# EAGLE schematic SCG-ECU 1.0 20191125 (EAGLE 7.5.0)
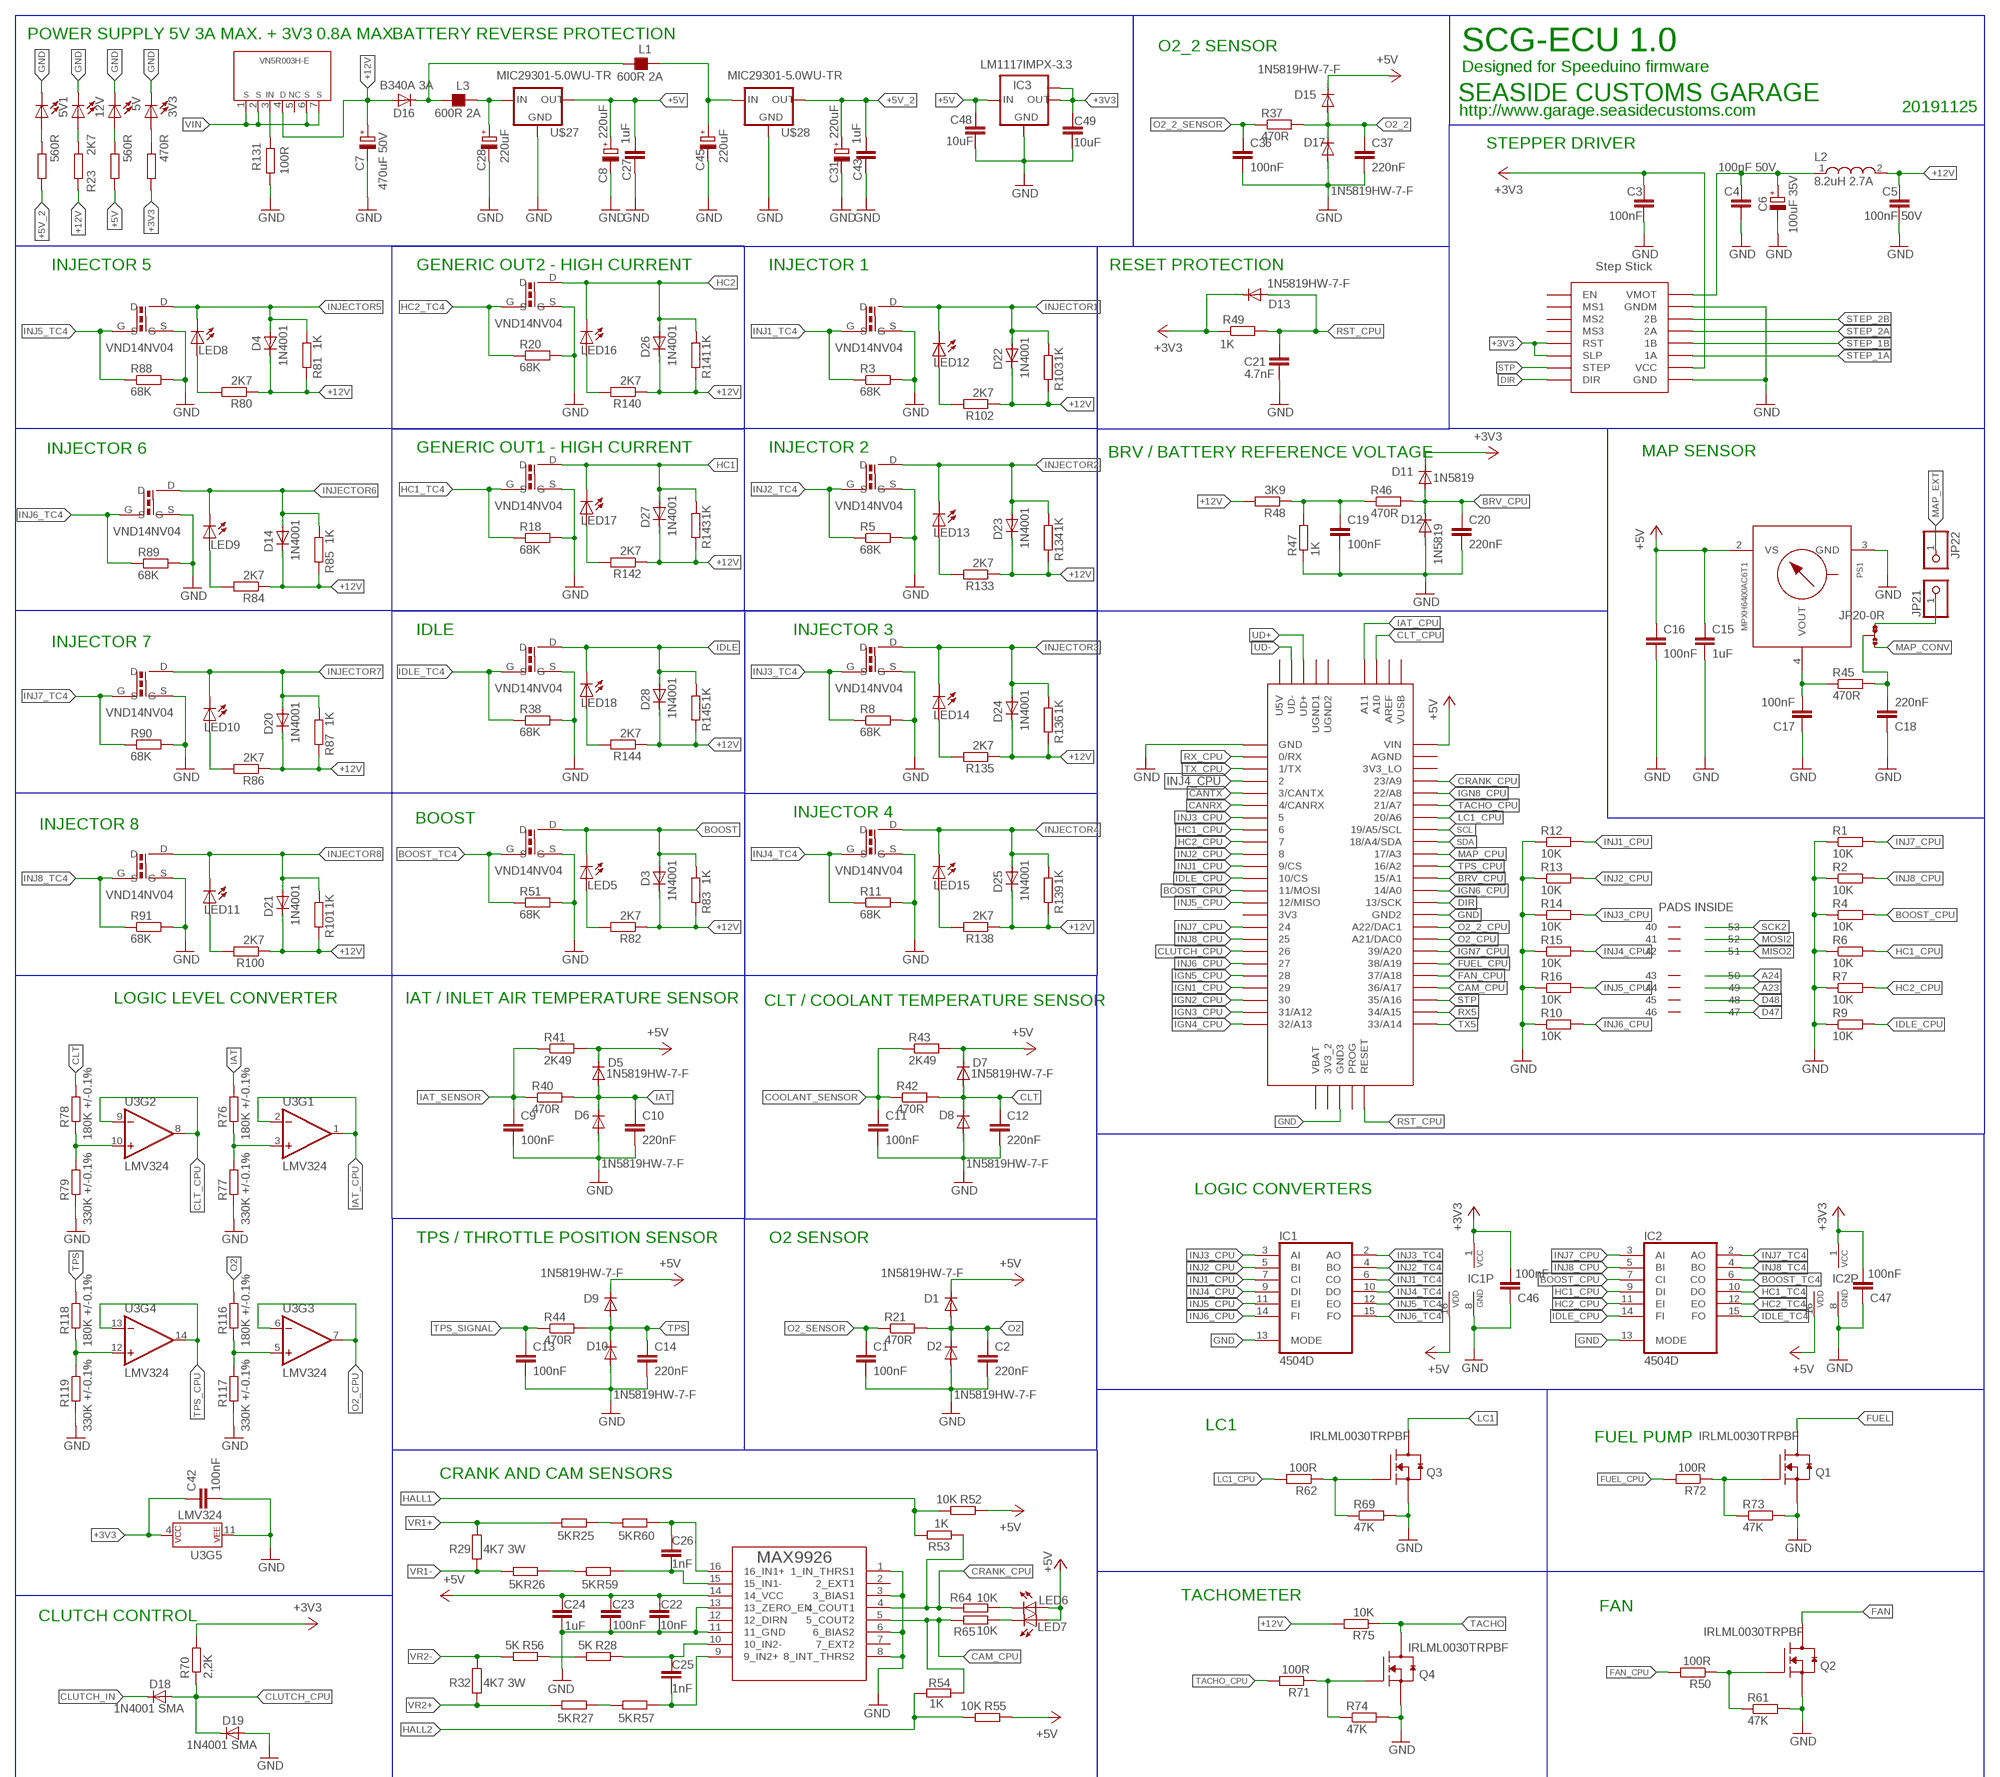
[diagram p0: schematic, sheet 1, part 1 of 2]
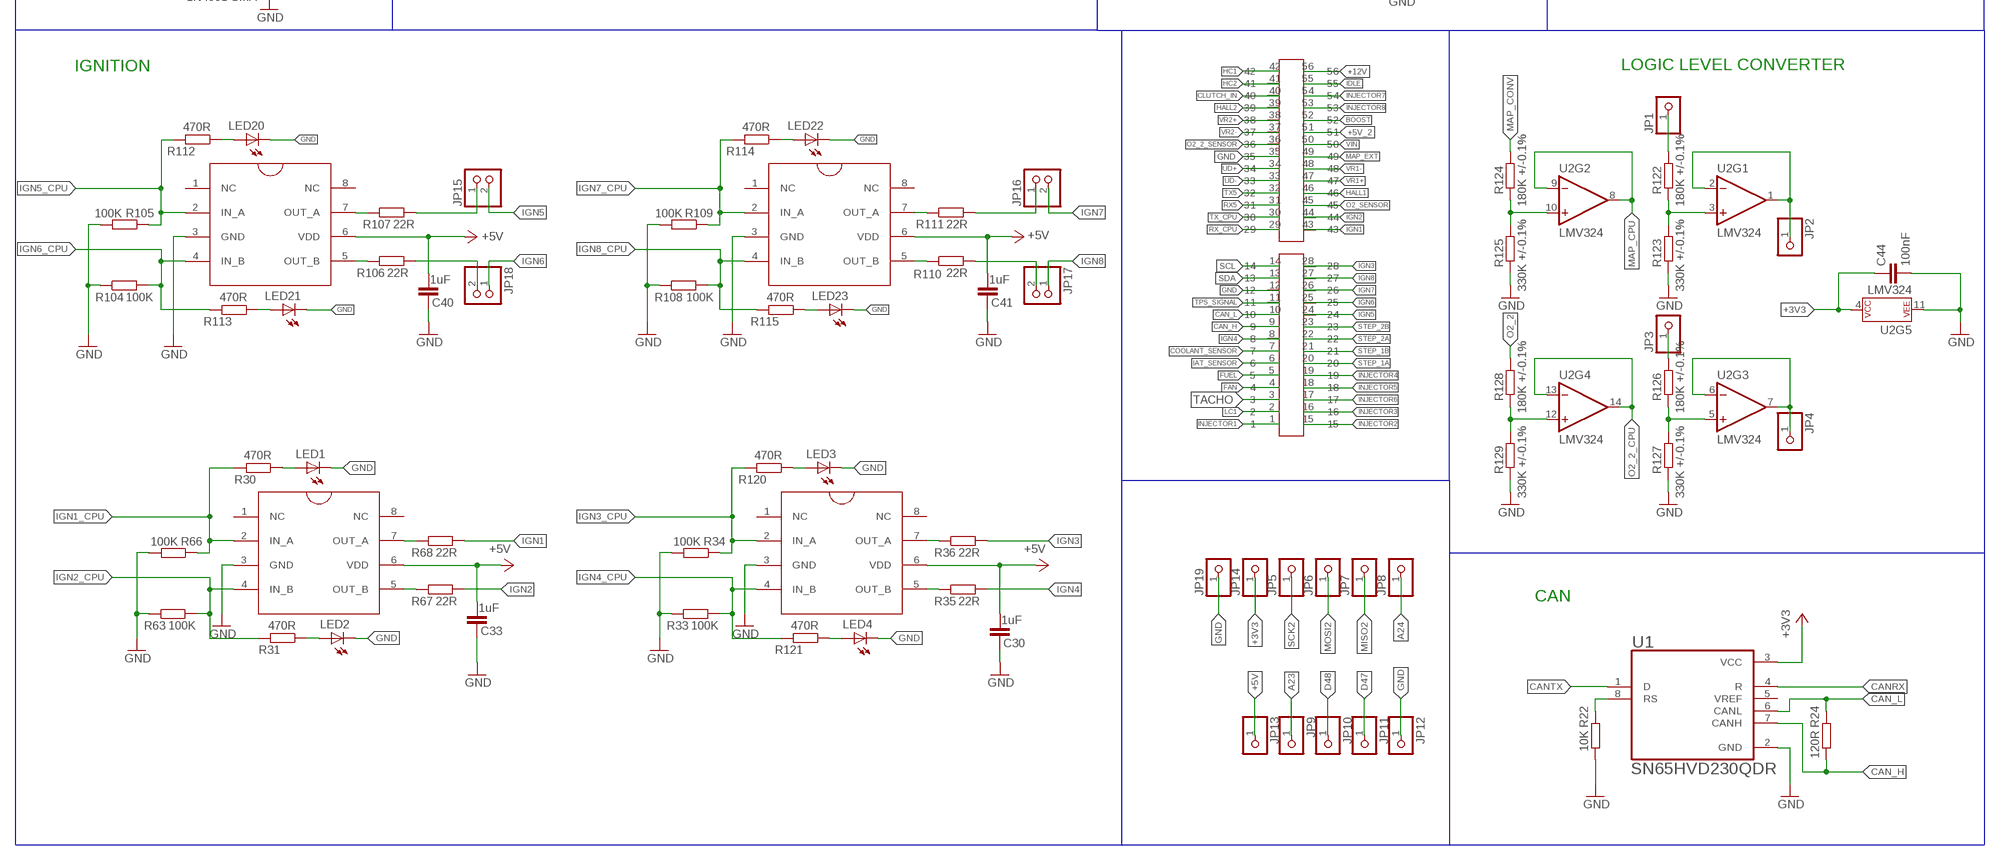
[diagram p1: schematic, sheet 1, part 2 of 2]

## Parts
3V3  LEDCHIP-LED0805  [CHIP-LED0805]
5V  LEDCHIP-LED0805  [CHIP-LED0805]
5V1  LEDCHIP-LED0805  [CHIP-LED0805]
12V  LEDCHIP-LED0805  [CHIP-LED0805]
C1  100nF  C-EUC0805  [C0805]
C2  220nF  C-EUC0805  [C0805]
C3  100nF  C-EUC0805  [C0805]
C4  100nF 50V  C-EUC0805  [C0805]
C5  100nF 50V  C-EUC0805  [C0805]
C6  100uF 35V  CPOL-EUD  [PANASONIC_D]
C7  470uF 50V  CPOL-EUG  [PANASONIC_G]
C8  220uF  CPOL-EUD  [PANASONIC_D]
C9  100nF  C-EUC0805  [C0805]
C10  220nF  C-EUC0805  [C0805]
C11  100nF  C-EUC0805  [C0805]
C12  220nF  C-EUC0805  [C0805]
C13  100nF  C-EUC0805  [C0805]
C14  220nF  C-EUC0805  [C0805]
C15  1uF  C-EUC0805  [C0805]
C16  100nF  C-EUC0805  [C0805]
C17  100nF  C-EUC0805  [C0805]
C18  220nF  C-EUC0805  [C0805]
C19  100nF  C-EUC0805  [C0805]
C20  220nF  C-EUC0805  [C0805]
C21  4.7nF  C-EUC0805  [C0805]
C22  10nF  C-EUC0805  [C0805]
C23  100nF  C-EUC0805  [C0805]
C24  1uF  C-EUC0805  [C0805]
C25  1nF  C-EUC0805  [C0805]
C26  1nF  C-EUC0805  [C0805]
C27  1uF  C-EUC0805  [C0805]
C28  220uF  CPOL-EUD  [PANASONIC_D]
C30  1uF  C-EUC0805  [C0805]
C31  220uF  CPOL-EUD  [PANASONIC_D]
C33  1uF  C-EUC0805  [C0805]
C36  100nF  C-EUC0805  [C0805]
C37  220nF  C-EUC0805  [C0805]
C40  1uF  C-EUC0805  [C0805]
C41  1uF  C-EUC0805  [C0805]
C42  100nF  C-EUC0805  [C0805]
C43  1uF  C-EUC0805  [C0805]
C44  100nF  C-EUC0805  [C0805]
C45  220uF  CPOL-EUD  [PANASONIC_D]
C46  100nF  C-EUC0805  [C0805]
C47  100nF  C-EUC0805  [C0805]
C48  10uF  C-EUC0805  [C0805]
C49  10uF  C-EUC0805  [C0805]
D1  1N5819HW-7-F  DIODE-SOD123  [SOD123]
D2  1N5819HW-7-F  DIODE-SOD123  [SOD123]
D3  1N4001  DIODE-D-2.5  [D-2.5]
D4  1N4001  DIODE-D-2.5  [D-2.5]
D5  1N5819HW-7-F  DIODE-SOD123  [SOD123]
D6  1N5819HW-7-F  DIODE-SOD123  [SOD123]
D7  1N5819HW-7-F  DIODE-SOD123  [SOD123]
D8  1N5819HW-7-F  DIODE-SOD123  [SOD123]
D9  1N5819HW-7-F  DIODE-SOD123  [SOD123]
D10  1N5819HW-7-F  DIODE-SOD123  [SOD123]
D11  1N5819  DIODE-SOD123  [SOD123]
D12  1N5819  DIODE-SOD123  [SOD123]
D13  1N5819HW-7-F  DIODE-SOD123  [SOD123]
D14  1N4001  DIODE-D-2.5  [D-2.5]
D15  1N5819HW-7-F  DIODE-SOD123  [SOD123]
D16  B340A 3A  S1A  [DO214AC]
D17  1N5819HW-7-F  DIODE-SOD123  [SOD123]
D18  1N4001 SMA  S1A  [DO214AC]
D19  1N4001 SMA  S1A  [DO214AC]
D20  1N4001  DIODE-D-2.5  [D-2.5]
D21  1N4001  DIODE-D-2.5  [D-2.5]
D22  1N4001  DIODE-D-2.5  [D-2.5]
D23  1N4001  DIODE-D-2.5  [D-2.5]
D24  1N4001  DIODE-D-2.5  [D-2.5]
D25  1N4001  DIODE-D-2.5  [D-2.5]
D26  1N4001  DIODE-D-2.5  [D-2.5]
D27  1N4001  DIODE-D-2.5  [D-2.5]
D28  1N4001  DIODE-D-2.5  [D-2.5]
IC1  4504D  [SO16]
IC2  4504D  [SO16]
IC3  LM1117IMPX-3.3  [SOT223]
JP1  PINHD-1X1  [1X01]
JP2  PINHD-1X1  [1X01]
JP3  PINHD-1X1  [1X01]
JP4  PINHD-1X1  [1X01]
JP5  PINHD-1X1  [1X01]
JP6  PINHD-1X1  [1X01]
JP7  PINHD-1X1  [1X01]
JP8  PINHD-1X1  [1X01]
JP9  PINHD-1X1  [1X01]
JP10  PINHD-1X1  [1X01]
JP11  PINHD-1X1  [1X01]
JP12  PINHD-1X1  [1X01]
JP13  PINHD-1X1  [1X01]
JP14  PINHD-1X1  [1X01]
JP15  PINHD-1X2  [1X02]
JP16  PINHD-1X2  [1X02]
JP17  PINHD-1X2  [1X02]
JP18  PINHD-1X2  [1X02]
JP19  PINHD-1X1  [1X01]
JP20  0R-JUMPA  [A0R-JMP]
JP21  PINHD-1X1  [1X01]
JP22  PINHD-1X1  [1X01]
L1  600R 2A  FB_1206  [L1206]
L2  8.2uH 2.7A  WE-PD_7332/7345_PLASTIC_BASE  [WE-PD_7332/7345_PLASTIC_BASE]
L3  600R 2A  FB_1206  [L1206]
LED1  LEDCHIP-LED0805  [CHIP-LED0805]
LED2  LEDCHIP-LED0805  [CHIP-LED0805]
LED3  LEDCHIP-LED0805  [CHIP-LED0805]
LED4  LEDCHIP-LED0805  [CHIP-LED0805]
LED5  LEDCHIPLED_0805  [CHIPLED_0805]
LED6  LEDCHIP-LED0805  [CHIP-LED0805]
LED7  LEDCHIP-LED0805  [CHIP-LED0805]
LED8  LEDCHIPLED_0805  [CHIPLED_0805]
LED9  LEDCHIPLED_0805  [CHIPLED_0805]
LED10  LEDCHIPLED_0805  [CHIPLED_0805]
LED11  LEDCHIPLED_0805  [CHIPLED_0805]
LED12  LEDCHIPLED_0805  [CHIPLED_0805]
LED13  LEDCHIPLED_0805  [CHIPLED_0805]
LED14  LEDCHIPLED_0805  [CHIPLED_0805]
LED15  LEDCHIPLED_0805  [CHIPLED_0805]
LED16  LEDCHIPLED_0805  [CHIPLED_0805]
LED17  LEDCHIPLED_0805  [CHIPLED_0805]
LED18  LEDCHIPLED_0805  [CHIPLED_0805]
LED20  LEDCHIP-LED0805  [CHIP-LED0805]
LED21  LEDCHIP-LED0805  [CHIP-LED0805]
LED22  LEDCHIP-LED0805  [CHIP-LED0805]
LED23  LEDCHIP-LED0805  [CHIP-LED0805]
PS1  MPXH6400AC6T1  [1317A]
Q1  IRLML0030TRPBF  MOSFET-NCH_SOT-23  [SOT95P280X135-3N]
Q2  IRLML0030TRPBF  MOSFET-NCH_SOT-23  [SOT95P280X135-3N]
Q3  IRLML0030TRPBF  MOSFET-NCH_SOT-23  [SOT95P280X135-3N]
Q4  IRLML0030TRPBF  MOSFET-NCH_SOT-23  [SOT95P280X135-3N]
R1  10K  R-EU_R0805  [R0805]
R2  10K  R-EU_R0805  [R0805]
R3  68K  R-EU_R0805  [R0805]
R4  10K  R-EU_R0805  [R0805]
R5  68K  R-EU_R0805  [R0805]
R6  10K  R-EU_R0805  [R0805]
R7  10K  R-EU_R0805  [R0805]
R8  68K  R-EU_R0805  [R0805]
R9  10K  R-EU_R0805  [R0805]
R10  10K  R-EU_R0805  [R0805]
R11  68K  R-EU_R0805  [R0805]
R12  10K  R-EU_R0805  [R0805]
R13  10K  R-EU_R0805  [R0805]
R14  10K  R-EU_R0805  [R0805]
R15  10K  R-EU_R0805  [R0805]
R16  10K  R-EU_R0805  [R0805]
R18  68K  R-EU_R0805  [R0805]
R20  68K  R-EU_R0805  [R0805]
R21  470R  R-EU_R0805  [R0805]
R22  10K  R-EU_R0805  [R0805]
R23  2K7  R-EU_R0805  [R0805]
R24  120R  R-EU_R0805  [R0805]
R25  5K  R-EU_R0805  [R0805]
R26  5K  R-EU_R0805  [R0805]
R27  5K  R-EU_R0805  [R0805]
R28  5K  R-EU_R0805  [R0805]
R29  4K7 3W  R-EU_R2512  [R2512]
R30  470R  R-EU_R0805  [R0805]
R31  470R  R-EU_R0805  [R0805]
R32  4K7 3W  R-EU_R2512  [R2512]
R33  100K  R-EU_R0805  [R0805]
R34  100K  R-EU_R0805  [R0805]
R35  22R  R-EU_M1206  [M1206]
R36  22R  R-EU_M1206  [M1206]
R37  470R  R-EU_R0805  [R0805]
R38  68K  R-EU_R0805  [R0805]
R40  470R  R-EU_R0805  [R0805]
R41  2K49  R-EU_R0805  [R0805]
R42  470R  R-EU_R0805  [R0805]
R43  2K49  R-EU_R0805  [R0805]
R44  470R  R-EU_R0805  [R0805]
R45  470R  R-EU_R0805  [R0805]
R46  470R  R-EU_R0805  [R0805]
R47  1K  R-EU_R0805  [R0805]
R48  3K9  R-EU_R0805  [R0805]
R49  1K  R-EU_R0805  [R0805]
R50  100R  R-EU_R0805  [R0805]
R51  68K  R-EU_R0805  [R0805]
R52  10K  R-EU_R0805  [R0805]
R53  1K  R-EU_R0805  [R0805]
R54  1K  R-EU_R0805  [R0805]
R55  10K  R-EU_R0805  [R0805]
R56  5K  R-EU_R0805  [R0805]
R57  5K  R-EU_R0805  [R0805]
R59  5K  R-EU_R0805  [R0805]
R60  5K  R-EU_R0805  [R0805]
R61  47K  R-EU_R0805  [R0805]
R62  100R  R-EU_R0805  [R0805]
R63  100K  R-EU_R0805  [R0805]
R64  10K  R-EU_R0805  [R0805]
R65  10K  R-EU_R0805  [R0805]
R66  100K  R-EU_R0805  [R0805]
R67  22R  R-EU_M1206  [M1206]
R68  22R  R-EU_M1206  [M1206]
R69  47K  R-EU_R0805  [R0805]
R70  2,2K  R-EU_R0805  [R0805]
R71  100R  R-EU_R0805  [R0805]
R72  100R  R-EU_R0805  [R0805]
R73  47K  R-EU_R0805  [R0805]
R74  47K  R-EU_R0805  [R0805]
R75  10K  R-EU_R0805  [R0805]
R76  180K +/-0.1%  R-EU_R0805  [R0805]
R77  330K +/-0.1%  R-EU_R0805  [R0805]
R78  180K +/-0.1%  R-EU_R0805  [R0805]
R79  330K +/-0.1%  R-EU_R0805  [R0805]
R80  2K7  R-EU_R0805  [R0805]
R81  1K  R-EU_R0805  [R0805]
R82  2K7  R-EU_R0805  [R0805]
R83  1K  R-EU_R0805  [R0805]
R84  2K7  R-EU_R0805  [R0805]
R85  1K  R-EU_R0805  [R0805]
R86  2K7  R-EU_R0805  [R0805]
R87  1K  R-EU_R0805  [R0805]
R88  68K  R-EU_R0805  [R0805]
R89  68K  R-EU_R0805  [R0805]
R90  68K  R-EU_R0805  [R0805]
R91  68K  R-EU_R0805  [R0805]
R100  2K7  R-EU_R0805  [R0805]
R101  1K  R-EU_R0805  [R0805]
R102  2K7  R-EU_R0805  [R0805]
R103  1K  R-EU_R0805  [R0805]
R104  100K  R-EU_R0805  [R0805]
R105  100K  R-EU_R0805  [R0805]
R106  22R  R-EU_M1206  [M1206]
R107  22R  R-EU_M1206  [M1206]
R108  100K  R-EU_R0805  [R0805]
R109  100K  R-EU_R0805  [R0805]
R110  22R  R-EU_M1206  [M1206]
R111  22R  R-EU_M1206  [M1206]
R112  470R  R-EU_R0805  [R0805]
R113  470R  R-EU_R0805  [R0805]
R114  470R  R-EU_R0805  [R0805]
R115  470R  R-EU_R0805  [R0805]
R116  180K +/-0.1%  R-EU_R0805  [R0805]
R117  330K +/-0.1%  R-EU_R0805  [R0805]
R118  180K +/-0.1%  R-EU_R0805  [R0805]
R119  330K +/-0.1%  R-EU_R0805  [R0805]
R120  470R  R-EU_R0805  [R0805]
R121  470R  R-EU_R0805  [R0805]
R122  180K +/-0.1%  R-EU_R0805  [R0805]
R123  330K +/-0.1%  R-EU_R0805  [R0805]
R124  180K +/-0.1%  R-EU_R0805  [R0805]
R125  330K +/-0.1%  R-EU_R0805  [R0805]
R126  180K +/-0.1%  R-EU_R0805  [R0805]
R127  330K +/-0.1%  R-EU_R0805  [R0805]
R128  180K +/-0.1%  R-EU_R0805  [R0805]
R129  330K +/-0.1%  R-EU_R0805  [R0805]
R130  560R  R-EU_R0805  [R0805]
R131  100R  R-EU_R0805  [R0805]
R132  560R  R-EU_R0805  [R0805]
R133  2K7  R-EU_R0805  [R0805]
R134  1K  R-EU_R0805  [R0805]
R135  2K7  R-EU_R0805  [R0805]
R136  1K  R-EU_R0805  [R0805]
R137  470R  R-EU_R0805  [R0805]
R138  2K7  R-EU_R0805  [R0805]
R139  1K  R-EU_R0805  [R0805]
R140  2K7  R-EU_R0805  [R0805]
R141  1K  R-EU_R0805  [R0805]
R142  2K7  R-EU_R0805  [R0805]
R143  1K  R-EU_R0805  [R0805]
R144  2K7  R-EU_R0805  [R0805]
R145  1K  R-EU_R0805  [R0805]
STEPSTICK-X  STEP-STICK  [STEP-STICK]
U1  SN65HVD230QDR  [SOIC127P600X175-8N]
U2  LMV324  [SO14]
U3  LMV324  [SO14]
U$1  TEENSY_3.5/3.6  [TEENSY_3.5/3.6]
U$2  DPAK_N-CHANNEL_MOSFET  [DPAK_N-CHANNEL_MOSFET]
U$3  DPAK_N-CHANNEL_MOSFET  [DPAK_N-CHANNEL_MOSFET]
U$4  DPAK_N-CHANNEL_MOSFET  [DPAK_N-CHANNEL_MOSFET]
U$5  DPAK_N-CHANNEL_MOSFET  [DPAK_N-CHANNEL_MOSFET]
U$6  DPAK_N-CHANNEL_MOSFET  [DPAK_N-CHANNEL_MOSFET]
U$8  DPAK_N-CHANNEL_MOSFET  [DPAK_N-CHANNEL_MOSFET]
U$9  TC427SO-8  [SO-8]
U$10  MAX9926  [QSOP16]
U$11  TC427SO-8  [SO-8]
U$12  DPAK_N-CHANNEL_MOSFET  [DPAK_N-CHANNEL_MOSFET]
U$13  DPAK_N-CHANNEL_MOSFET  [DPAK_N-CHANNEL_MOSFET]
U$17  56PIN_CONNECTOR  [56PIN_CONNECTOR]
U$18  VN5R003H-E  [VN5R003H-E_HPAK_TO267_7]
U$19  DPAK_N-CHANNEL_MOSFET  [DPAK_N-CHANNEL_MOSFET]
U$20  DPAK_N-CHANNEL_MOSFET  [DPAK_N-CHANNEL_MOSFET]
U$21  DPAK_N-CHANNEL_MOSFET  [DPAK_N-CHANNEL_MOSFET]
U$22  DPAK_N-CHANNEL_MOSFET  [DPAK_N-CHANNEL_MOSFET]
U$25  TC427SO-8  [SO-8]
U$26  TC427SO-8  [SO-8]
U$27  MIC29301-5.0WU-TR  [TO263-3]
U$28  MIC29301-5.0WU-TR  [TO263-3]

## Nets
+3V3: C3.1 C42.1 C44.1 C46.2 C47.2 C49.1 D11.C D13.C IC1.1(VCC) IC2.1(VCC) IC3.2(OUT) IC3.TAB(OUT1) JP14.1 R49.1 R70.2 R137.2 STEPSTICK-X.RST STEPSTICK-X.SLP STEPSTICK-X.VCC U1.3(VCC) U2.4(P$V+) U3.4(P$V+)
+5V: C8.+ C15.1 C16.1 C22.1 C23.1 C24.1 C27.1 C30.2 C33.2 C40.2 C41.2 C48.1 D1.C D5.C D7.C D9.C D15.C IC1.16(VDD) IC2.16(VDD) IC3.3(IN) JP13.1 LED6.A LED7.A PS1.2(VS) R41.2 R43.2 R52.1 R55.1 R130.2 U$1.VIN U$9.6(VDD) U$10.14(14_VCC) U$11.6(VDD) U$25.6(VDD) U$26.6(VDD) U$27.3(OUT)
+5V_2: C31.+ C43.1 R132.2 U$17.51 U$28.3(OUT)
+12V: C5.1 C7.+ D3.C D4.C D14.C D16.A D20.C D21.C D22.C D23.C D24.C D25.C D26.C D27.C D28.C L2.2 R23.2 R48.2 R75.2 R80.1 R81.1 R82.1 R83.1 R84.1 R85.1 R86.1 R87.1 R100.1 R101.1 R102.1 R103.1 R133.1 R134.1 R135.1 R136.1 R138.1 R139.1 R140.1 R141.1 R142.1 R143.1 R144.1 R145.1 U$17.56 U$18.4
A23: JP9.1 U$1.49
A24: JP8.1 U$1.50
BOOST: D3.A LED5.C R83.2 U$13.D U$17.52
BOOST_CPU: IC2.7(CI) R4.2 U$1.11/MOSI
BOOST_TC4: IC2.6(CO) R51.1 U$13.G
BRV_CPU: C20.1 D11.A D12.C R46.2 U$1.15/A1
CAM_CPU: R54.1 R65.1 U$1.36/A17 U$10.5(5_COUT2)
CAN_H: R24.2 U1.7(CANH) U$17.9
CAN_L: R24.1 U1.6(CANL) U$17.10
CANRX: U1.4(R) U$1.4/CANRX
CANTX: U1.1(D) U$1.3/CANTX
CLT: C12.1 D7.A D8.C R42.2 R78.2
CLT_CPU: U3.8(OUT) U3.9(-IN) U$1.A10
CLUTCH_CPU: D18.A D19.C R70.1 U$1.26
CLUTCH_IN: D18.C U$17.40
COOLANT_SENSOR: C11.1 R42.1 R43.1 U$17.7
CRANK_CPU: R53.2 R64.1 U$1.23/A9 U$10.4(4_COUT1)
D47: JP11.1 U$1.47
D48: JP10.1 U$1.48
DIR: STEPSTICK-X.DIR U$1.13/SCK
FAN: Q2.3(D) U$17.4
FAN_CPU: R50.2 U$1.37/A18
FUEL: Q1.3(D) U$17.5
FUEL_CPU: R72.2 U$1.38/A19
GND: 3V3.C 5V1.C 5V.C 12V.C C1.2 C2.2 C3.2 C4.2 C5.2 C6.- C7.- C8.- C9.2 C10.2 C11.2 C12.2 C13.2 C14.2 C15.2 C16.2 C17.1 C18.1 C19.2 C20.2 C21.2 C22.2 C23.2 C24.2 C27.2 C28.- C30.1 C31.- C33.1 C36.2 C37.2 C40.1 C41.1 C42.2 C43.2 C44.2 C45.- C46.1 C47.1 C48.2 C49.2 D2.A D6.A D8.A D10.A D12.A D17.A D19.A IC1.8(GND) IC1.13(MODE) IC2.8(GND) IC2.13(MODE) IC3.1(GND) JP12.1 JP19.1 LED1.C LED2.C LED3.C LED4.C LED20.C LED21.C LED22.C LED23.C PS1.3(GND) Q1.2(S) Q2.2(S) Q3.2(S) Q4.2(S) R1.1 R2.1 R3.2 R4.1 R5.2 R6.1 R7.1 R8.2 R9.1 R10.1 R11.2 R12.1 R13.1 R14.1 R15.1 R16.1 R18.2 R20.2 R22.2 R33.1 R34.2 R38.2 R47.1 R51.2 R61.2 R63.1 R66.2 R69.2 R73.2 R74.2 R77.1 R79.1 R88.2 R89.2 R90.2 R91.2 R104.1 R105.2 R108.1 R109.2 R117.1 R119.1 R123.1 R125.1 R127.1 R129.1 R131.1 STEPSTICK-X.GND STEPSTICK-X.GNDM U1.2(GND) U2.11(P$V-) U3.11(P$V-) U$1.GND U$1.GND2 U$1.GND3 U$2.S U$3.S U$4.S U$5.S U$6.S U$8.S U$9.3(GND) U$10.1(1_IN_THRS1) U$10.3(3_BIAS1) U$10.6(6_BIAS2) U$10.8(8_INT_THRS2) U$10.11(11_GND) U$10.13(13_ZERO_EN) U$11.3(GND) U$12.S U$13.S U$17.12 U$17.35 U$19.S U$20.S U$21.S U$22.S U$25.3(GND) U$26.3(GND) U$27.TAB(GND) U$28.TAB(GND)
HALL1: R52.2 R53.1 U$17.46
HALL2: R54.2 R55.2 U$17.39
HC1: D27.A LED17.C R143.2 U$3.D U$17.42
HC1_CPU: IC2.9(DI) R6.2 U$1.6
HC1_TC4: IC2.10(DO) R18.1 U$3.G
HC2: D26.A LED16.C R141.2 U$2.D U$17.41
HC2_CPU: IC2.11(EI) R7.2 U$1.7
HC2_TC4: IC2.12(EO) R20.1 U$2.G
IAT: C10.1 D5.A D6.C R40.2 R76.2
IAT_CPU: U3.1(OUT) U3.2(-IN) U$1.A11
IAT_SENSOR: C9.1 R40.1 R41.1 U$17.6
IDLE: D28.A LED18.C R145.2 U$5.D U$17.55
IDLE_CPU: IC2.14(FI) R9.2 U$1.10/CS
IDLE_TC4: IC2.15(FO) R38.1 U$5.G
IGN1: R68.2 U$17.43
IGN1_CPU: R30.2 R66.1 U$1.29 U$9.2(IN_A)
IGN2: R67.2 U$17.44
IGN2_CPU: R31.2 R63.2 U$1.30 U$9.4(IN_B)
IGN3: R36.2 U$17.28
IGN3_CPU: R34.1 R120.2 U$1.31/A12 U$11.2(IN_A)
IGN4: R35.2 U$17.8
IGN4_CPU: R33.2 R121.2 U$1.32/A13 U$11.4(IN_B)
IGN5: JP15.2 U$17.24
IGN5_CPU: R105.1 R112.2 U$1.28 U$25.2(IN_A)
IGN6: JP18.1 U$17.25
IGN6_CPU: R104.2 R113.2 U$1.14/A0 U$25.4(IN_B)
IGN7: JP16.2 U$17.26
IGN7_CPU: R109.1 R114.2 U$1.39/A20 U$26.2(IN_A)
IGN8: JP17.1 U$17.27
IGN8_CPU: R108.2 R115.2 U$1.22/A8 U$26.4(IN_B)
INJ1_CPU: IC1.7(CI) R12.2 U$1.9/CS
INJ1_TC4: IC1.6(CO) R3.1 U$12.G
INJ2_CPU: IC1.5(BI) R13.2 U$1.8
INJ2_TC4: IC1.4(BO) R5.1 U$4.G
INJ3_CPU: IC1.3(AI) R14.2 U$1.5
INJ3_TC4: IC1.2(AO) R8.1 U$6.G
INJ4_CPU: IC1.9(DI) R15.2 U$1.2
INJ4_TC4: IC1.10(DO) R11.1 U$8.G
INJ5_CPU: IC1.11(EI) R16.2 U$1.12/MISO
INJ5_TC4: IC1.12(EO) R88.1 U$19.G
INJ6_CPU: IC1.14(FI) R10.2 U$1.27
INJ6_TC4: IC1.15(FO) R89.1 U$20.G
INJ7_CPU: IC2.3(AI) R1.2 U$1.24
INJ7_TC4: IC2.2(AO) R90.1 U$21.G
INJ8_CPU: IC2.5(BI) R2.2 U$1.25
INJ8_TC4: IC2.4(BO) R91.1 U$22.G
INJECTOR1: D22.A LED12.C R103.2 U$12.D U$17.1
INJECTOR2: D23.A LED13.C R134.2 U$4.D U$17.15
INJECTOR3: D24.A LED14.C R136.2 U$6.D U$17.16
INJECTOR4: D25.A LED15.C R139.2 U$8.D U$17.19
INJECTOR5: D4.A LED8.C R81.2 U$17.18 U$19.D
INJECTOR6: D14.A LED9.C R85.2 U$17.17 U$20.D
INJECTOR7: D20.A LED10.C R87.2 U$17.54 U$21.D
INJECTOR8: D21.A LED11.C R101.2 U$17.53 U$22.D
LC1: Q3.3(D) U$17.2
LC1_CPU: R62.2 U$1.20/A6
MAP_CONV: JP20.1 R124.2
MAP_CPU: U2.8(OUT) U2.9(-IN) U$1.17/A3
MAP_EXT: JP22.1 U$17.49
MISO2: JP7.1 U$1.51
MOSI2: JP6.1 U$1.52
N$1: LED8.A R80.2
N$2: LED5.A R82.2
N$3: R67.1 U$9.5(OUT_B)
N$5: R68.1 U$9.7(OUT_A)
N$6: R35.1 U$11.5(OUT_B)
N$8: R36.1 U$11.7(OUT_A)
N$9: Q2.1(G) R50.1 R61.1
N$11: Q3.1(G) R62.1 R69.1
N$12: R22.1 U1.8(RS)
N$13: R78.1 R79.2 U3.10(+IN)
N$15: R76.1 R77.2 U3.3(+IN)
N$16: LED1.A R30.1
N$17: R116.1 R117.2 U3.5(+IN)
N$18: LED9.A R84.2
N$19: C4.1 C6.+ L2.1 STEPSTICK-X.VMOT
N$20: LED11.A R100.2
N$21: LED15.A R138.2
N$22: LED10.A R86.2
N$25: LED2.A R31.1
N$27: C19.1 R46.1 R47.2 R48.1
N$29: Q4.1(G) R71.1 R74.1
N$31: LED12.A R102.2
N$32: C17.2 PS1.4(VOUT) R45.1
N$34: LED16.A R140.2
N$35: C25.2 R57.1 U$10.9(9_IN2+)
N$36: C26.1 R60.1 U$10.16(16_IN1+)
N$37: C26.2 R59.1 U$10.15(15_IN1-)
N$38: C25.1 R28.1 U$10.10(10_IN2-)
N$39: R106.1 U$25.5(OUT_B)
N$40: R107.1 U$25.7(OUT_A)
N$41: R25.1 R60.2
N$42: R110.1 U$26.5(OUT_B)
N$43: R111.1 U$26.7(OUT_A)
N$44: LED20.A R112.1
N$45: LED21.A R113.1
N$46: LED22.A R114.1
N$47: LED23.A R115.1
N$49: LED7.C R65.2
N$50: LED6.C R64.2
N$51: 12V.A R23.1
N$54: 5V.A R130.1
N$55: R26.1 R59.2
N$56: R27.1 R57.2
N$57: R28.2 R56.1
N$58: R122.1 R123.2 U2.3(+IN)
N$59: R118.1 R119.2 U3.12(+IN)
N$65: R124.1 R125.2 U2.10(+IN)
N$66: R126.1 R127.2 U2.5(+IN)
N$67: R128.1 R129.2 U2.12(+IN)
N$68: JP1.1 R122.2
N$69: JP2.1 U2.1(OUT) U2.2(-IN)
N$70: JP3.1 R126.2
N$71: JP4.1 U2.6(-IN) U2.7(OUT)
N$72: LED3.A R120.1
N$73: LED4.A R121.1
N$74: R131.2 U$18.3
N$75: D16.C L1.2 L3.2
N$76: C45.+ L1.1 U$28.1(IN)
N$77: 5V1.A R132.1
N$78: C28.+ L3.1 U$27.1(IN)
N$79: LED13.A R133.2
N$81: 3V3.A R137.1
N$83: LED14.A R135.2
N$84: LED17.A R142.2
N$87: LED18.A R144.2
N$91: Q1.1(G) R72.1 R73.1
N$326: JP15.1 R107.2
N$327: JP16.1 R111.2
N$328: JP18.2 R106.2
N$329: JP17.2 R110.2
N$338: JP20.3 JP21.1
N$339: C18.2 JP20.2 R45.2
O2: C2.1 D1.A D2.C R21.2 R116.2
O2_2: C37.1 D15.A D17.C R37.2 R128.2
O2_2_CPU: U2.13(-IN) U2.14(OUT) U$1.A22/DAC1
O2_2_SENSOR: C36.1 R37.1 U$17.36
O2_CPU: U3.6(-IN) U3.7(OUT) U$1.21/DAC0(A21/DAC0)
O2_SENSOR: C1.1 R21.1 U$17.45
RST_CPU: C21.1 D13.A R49.2 U$1.RESET
RX5: U$1.34/A15 U$17.31
RX_CPU: U$1.0/RX U$17.29
SCK2: JP5.1 U$1.53
SCL: U$1.19/A5/SCL U$17.14
SDA: U$1.18/A4/SDA U$17.13
STEP_1A: STEPSTICK-X.1A U$17.20
STEP_1B: STEPSTICK-X.1B U$17.21
STEP_2A: STEPSTICK-X.2A U$17.22
STEP_2B: STEPSTICK-X.2B U$17.23
STP: STEPSTICK-X.SPT(STEP) U$1.35/A16
TACHO: Q4.3(D) R75.1 U$17.3
TACHO_CPU: R71.2 U$1.21/A7
TPS: C14.1 D9.A D10.C R44.2 R118.2
TPS_CPU: U3.13(-IN) U3.14(OUT) U$1.16/A2
TPS_SIGNAL: C13.1 R44.1 U$17.11
TX5: U$1.33/A14 U$17.32
TX_CPU: U$1.1/TX U$17.30
UD+: U$1.UD+ U$17.34
UD-: U$1.UD- U$17.33
VIN: U$17.50 U$18.1 U$18.2 U$18.6 U$18.7
VR1+: R25.2 R29.1 U$17.47
VR1-: R26.2 R29.2 U$17.48
VR2+: R27.2 R32.2 U$17.38
VR2-: R32.1 R56.2 U$17.37
Unconnected: PS1.1(NC) PS1.5(NC) PS1.6(NC) STEPSTICK-X.EN STEPSTICK-X.MS1 STEPSTICK-X.MS2 STEPSTICK-X.MS3 U1.5(VREF) U$1.3V3 U$1.3V3_2 U$1.3V3_LO U$1.40 U$1.41 U$1.42 U$1.43 U$1.44 U$1.45 U$1.46 U$1.AGND U$1.AREF U$1.PROG U$1.U5V U$1.UGND1 U$1.UGND2 U$1.VBAT U$1.VUSB U$9.1(NC) U$9.8(NC) U$10.2(2_EXT1) U$10.7(7_EXT2) U$10.12(12_DIRN) U$11.1(NC) U$11.8(NC) U$18.5 U$25.1(NC) U$25.8(NC) U$26.1(NC) U$26.8(NC)

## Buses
B$1

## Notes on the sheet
- POWER SUPPLY 5V 3A MAX. + 3V3 0.8A MAX. | BATTERY REVERSE PROTECTION
- O2_2 SENSOR | SCG-ECU 1.0
- Designed for Speeduino firmware
- SEASIDE CUSTOMS GARAGE
- http://www.garage.seasidecustoms.com | 20191125
- STEPPER DRIVER
- INJECTOR 5 | GENERIC OUT2 - HIGH CURRENT | INJECTOR 1 | RESET PROTECTION
- INJECTOR 6 | GENERIC OUT1 - HIGH CURRENT | INJECTOR 2 | MAP SENSOR
- BRV / BATTERY REFERENCE VOLTAGE
- IDLE | INJECTOR 3
- INJECTOR 7
- INJECTOR 4
- BOOST
- INJECTOR 8
- LOGIC LEVEL CONVERTER | IAT / INLET AIR TEMPERATURE SENSOR | CLT / COOLANT TEMPERATURE SENSOR
- LOGIC CONVERTERS
- TPS / THROTTLE POSITION SENSOR | O2 SENSOR
- LC1
- FUEL PUMP
- CRANK AND CAM SENSORS
- TACHOMETER
- FAN
- CLUTCH CONTROL
- IGNITION | LOGIC LEVEL CONVERTER
- CAN

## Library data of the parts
3V3 5V 5V1 12V LED1-LED18 LED20-LED23 = led:LED: LED
C1-C5 C9-C27 C30 C33 C36 C37 C40-C44 C46-C49 = resistor:C-EU: CAPACITOR, European symbol
C6-C8 C28 C31 C45 = resistor:CPOL-EU: POLARIZED CAPACITOR, European symbol
D1-D15 D17 D20-D28 = diode:DIODE-: DIODE
D16 D18 D19 = DO-214AC:S1*: S1A - S1M General Purpose Rectifiers; MF: Fairchild; MPN: S1A; OC_FARNELL: 9843868; OC_NEWARK: 58K9551
IC1 IC2 = 45xx:4504: TTL or CMOS to CMOS hex LEVEL SHIFTER
IC3 = lm1117:LM1117IMPX-*
JP1-JP14 JP19 JP21 JP22 = pinhead:PINHD-1X1: PIN HEADER
JP15-JP18 = pinhead:PINHD-1X2: PIN HEADER
JP20 = jump-0r-smd:0R-JUMP: SMD 0R 0805 Jumper
L1 L3 = rc-master-smd:FB_: FERRITE BEAD
L2 = Wurth Passive:WE-PD: SMD Shielded Power Inductor
PS1 = mpx-freescale:MPXH6400A: High Temperature Accuracy Integrated Silicon Pressure Sensor for Measuring Absolute Pressure, On-Chip Signal Conditioned, Temperature Compensated and Calibrated INTEGRATED PRESSURE SENSOR 20 TO 400 kPA (3.0 TO 58 psi) 0.2 TO 4.8 V OUTPUT (3.0 TO 58 psi)
Q1-Q4 = ipc-7351-transistor:MOSFET-NCH_
R1-R16 R18 R20-R38 R40-R57 R59-R91 R100-R145 = resistor:R-EU_: RESISTOR, European symbol
STEPSTICK-X = Arduino library Stepstick:STEP-STICK
U1 = SN65HVD230QDR:SN65HVD230QDR: Automotive Catalog 3.3-V CAN Transceivers 8-SOIC -40 to 125; AVAILABILITY: Good; DESCRIPTION: Automotive Catalog 3.3-V CAN Transceivers 8-SOIC -40 to 125; MF: Texas Instruments; MP: SN65HVD230QDR; PACKAGE: SOIC-8 Texas Instruments; PRICE: 1.62 USD
U2 U3 = SparkFun-IC-Amplifiers:LMV324: IC LMV324 Quad Op Amp Jellybean quad op-amp Datasheet SparkFun Products SparkFun Sensor Kit (DEV-13754) SparkFun Inventor's Kit for Arduino 101 (KIT-13844) SparkFun Sound Detector (SEN-12642); PROD_ID: IC-08227
U$1 = Teensy356_full_basic:TEENSY_3.5/3.6
U$2-U$6 U$8 U$12 U$13 U$19-U$22 = VND14NV04:DPAK_N-CHANNEL_MOSFET: VND14NV04
U$9 U$11 U$25 U$26 = TC426,427,428:TC427
U$10 = max9926:MAX9926
U$17 = 56pin_connector:56PIN_CONNECTOR
U$18 = VN5R003H-E - HPAK:VN5R003H-E
U$27 U$28 = MIC29301-5.0WU-TR - regulator 5V liniowy 3A:MIC29301-5.0WU-TR

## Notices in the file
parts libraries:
Wurth Passive: Copyright: Würth Elektronik
SparkFun-IC-Amplifiers: Licensing: Creative Commons ShareAlike 4.0 International - https://creativecommons.org/licenses/by-sa/4.0
rc-master-smd: Copyright (C) 2007, Bob Starr
